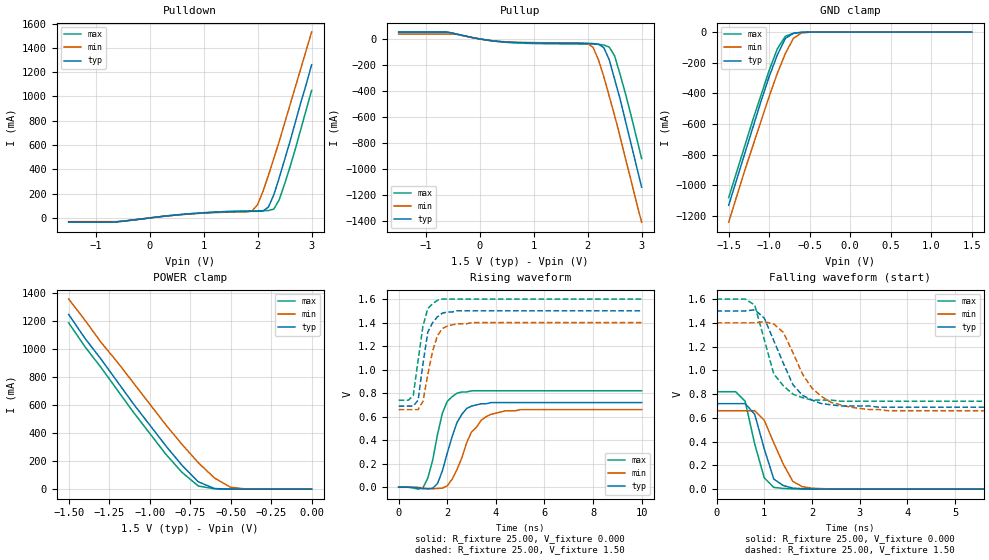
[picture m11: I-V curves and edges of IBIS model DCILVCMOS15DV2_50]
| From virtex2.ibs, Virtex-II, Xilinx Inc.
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|   Model DCILVCMOS15DV2_50
[Model]   DCILVCMOS15DV2_50
Model_type   I/O
Polarity   Non-Inverting
Enable   Active-Low
Vinh = 1.05V
Vinl = 0.3V
Vmeas =   0.75V
Cref =  0pF
Rref =   1.00M
Vref =  0.000V
C_comp   10.00pF   10.00pF   10.00pF
[Temperature Range]   25.00   100.00   0.000
[Voltage Range]   1.50V   1.40V   1.60V
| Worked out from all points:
|   slope of the pulldown table from 0 to 0.225 V, typ, clamps not added: 18.4 ohm
|   slope of the pullup table from 0 to 0.225 V, typ, clamps not added: 16.4 ohm
|   GND clamp passes 1 mA (typ) near -0.57 V on its own axis
|   POWER clamp passes 1 mA (typ) near -0.52 V on its own axis
|   rising waveform, R_fixture 25.00, V_fixture 0.000: 20-80 % time 669ps typ, 904ps min, 539ps max; typ from 0 V to 0.72 V
|   rising waveform, R_fixture 25.00, V_fixture 1.50: 20-80 % time 373ps typ, 474ps min, 389ps max; typ from 0.69 V to 1.5 V
|   falling waveform, R_fixture 25.00, V_fixture 0.000: 20-80 % time 316ps typ, 453ps min, 305ps max; typ from 0.72 V to 0 V
|   falling waveform, R_fixture 25.00, V_fixture 1.50: 20-80 % time 555ps typ, 640ps min, 432ps max; typ from 1.5 V to 0.69 V
[Pulldown]
| voltage   I(typ)   I(min)   I(max)
-1.5V     -34.98mA   -30.6mA    -34.01mA
-600mV    -31.87mA   -30.6mA    -30.85mA
700mV     32.61mA    31.18mA    32.91mA
1.9V      54.06mA    58.57mA    58.51mA
2V        54.49mA    110mA      58.88mA
2.1V      57.04mA    220mA      59.29mA
2.2V      89.88mA    350mA      60.89mA
2.3V      190mA      490mA      72.66mA
2.4V      330mA      630mA      150mA
2.5V      480mA      780mA      280mA
2.7V      790mA      1.08A      570mA
3V        1.26A      1.53A      1.05A
[Pullup]
| voltage   I(typ)   I(min)   I(max)
-1.5V     52.69mA    37.58mA    52.16mA
-500mV    45.15mA    37.58mA    43.69mA
400mV     -21.22mA   -19.97mA   -22.83mA
1.9V      -33.89mA   -31.85mA   -39.31mA
2V        -34.2mA    -35.85mA   -39.59mA
2.1V      -35.36mA   -64.05mA   -39.93mA
2.2V      -40.65mA   -160mA     -41.2mA
2.3V      -66.86mA   -290mA     -46.91mA
2.4V      -160mA     -440mA     -62.28mA
2.5V      -310mA     -590mA     -130mA
2.7V      -630mA     -920mA     -420mA
3V        -1.14A     -1.41A     -920mA
[GND_clamp]
| voltage   I(typ)   I(min)   I(max)
-1.5V     -1.13A     -1.24A     -1.08A
-1.3V     -790mA     -900mA     -740mA
-1.2V     -620mA     -740mA     -570mA
-1.1V     -450mA     -580mA     -410mA
-1V       -290mA     -420mA     -250mA
-900mV    -150mA     -270mA     -110mA
-800mV    -40.96mA   -140mA     -27.15mA
-700mV    -7.52mA    -40.16mA   -8.06mA
-600mV    -1.38mA    -5.56mA    -1.57mA
-500mV    -120uA     -650uA     -120uA
1.5V      27.96pA    98.69nA    16.96pA
[POWER_clamp]
| voltage   I(typ)   I(min)   I(max)
-1.5V     1.25A      1.36A      1.19A
-1.4V     1.08A      1.21A      1.02A
-1.3V     930mA      1.05A      870mA
-1.2V     770mA      910mA      710mA
-1.1V     610mA      760mA      550mA
-900mV    310mA      460mA      250mA
-800mV    170mA      320mA      120mA
-700mV    52.75mA    190mA      22.81mA
-600mV    4.57mA     79.88mA    2.44mA
-500mV    270uA      13.45mA    250uA
-400mV    16.38uA    820uA      14.46uA
0V        27.96pA    880pA      24.27pA
[Ramp]
| variable   typ   min   max
dV/dt_r   0.43/0.66n   0.40/0.89n   0.49/0.50n
dV/dt_f   0.48/0.47n   0.45/0.61n   0.52/0.38n
R_load = 25.00
[Rising Waveform]
R_fixture = 25.00
V_fixture = 0.000
| time   V(typ)   V(min)   V(max)
0s        0V         0V         0V
1ns       -12.98mV   -6.87mV    -4.96mV
1.2ns     -12.77mV   -12.73mV   78.26mV
1.6ns     32.68mV    -10.73mV   450mV
1.8ns     140mV      -7.2mV     630mV
2ns       290mV      11.71mV    730mV
2.4ns     550mV      150mV      800mV
3ns       690mV      470mV      820mV
3.8ns     720mV      620mV      820mV
10ns      720mV      660mV      820mV
[Rising Waveform]
R_fixture = 25.00
V_fixture = 1.50
V_fixture_min = 1.40
V_fixture_max = 1.60
| time   V(typ)   V(min)   V(max)
0s        690mV      660mV      740mV
600ps     690mV      660mV      780mV
800ps     740mV      660mV      1.08V
1ns       1.05V      730mV      1.37V
1.2ns     1.32V      960mV      1.52V
1.4ns     1.4V       1.16V      1.56V
1.6ns     1.45V      1.29V      1.59V
2ns       1.49V      1.37V      1.6V
3ns       1.5V       1.4V       1.6V
10ns      1.5V       1.4V       1.6V
[Falling Waveform]
R_fixture = 25.00
V_fixture = 0.000
| time   V(typ)   V(min)   V(max)
0s        720mV      660mV      820mV
400ps     720mV      660mV      820mV
600ps     720mV      660mV      740mV
800ps     630mV      660mV      380mV
1ns       340mV      580mV      95.85mV
1.2ns     84.67mV    390mV      14.95mV
1.4ns     30.06mV    210mV      6.1mV
1.6ns     8.93mV     65.1mV     2.42mV
2ns       2.04mV     8.39mV     610uV
10ns      4.26uV     -26.72uV   10.47uV
[Falling Waveform]
R_fixture = 25.00
V_fixture = 1.50
V_fixture_min = 1.40
V_fixture_max = 1.60
| time   V(typ)   V(min)   V(max)
0s        1.5V       1.4V       1.6V
800ps     1.51V      1.4V       1.55V
1ns       1.44V      1.41V      1.26V
1.2ns     1.25V      1.39V      970mV
1.4ns     1.06V      1.32V      870mV
1.6ns     880mV      1.15V      800mV
2ns       750mV      850mV      750mV
2.4ns     710mV      730mV      750mV
3.6ns     690mV      660mV      740mV
10ns      690mV      660mV      740mV
